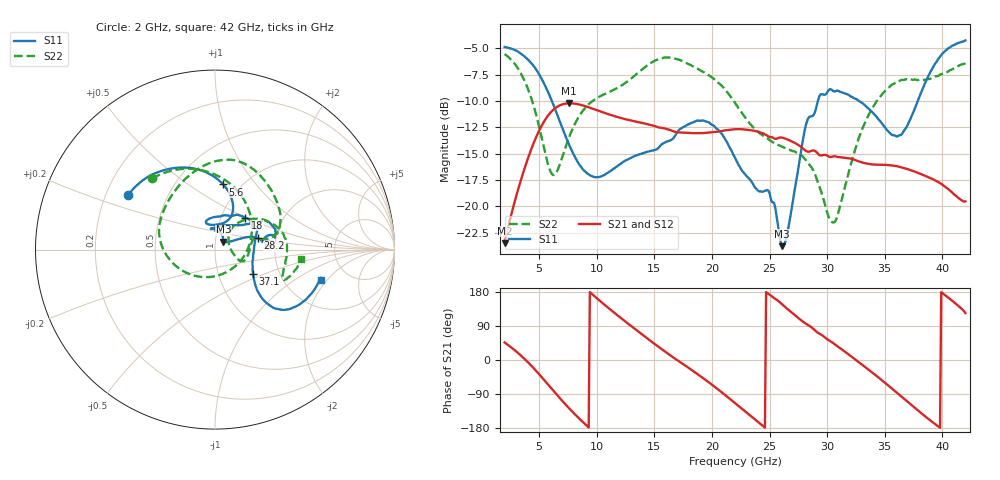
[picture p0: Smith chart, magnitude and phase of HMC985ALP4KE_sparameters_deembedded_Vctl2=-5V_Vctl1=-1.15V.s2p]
!s2p File: Measurements: S11, S21, S12, S22
# GHz S dB R 50.0
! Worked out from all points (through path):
!   401 points, 2 GHz to 42 GHz, reference 50 ohm
!   highest |S21| = -10.21 dB at 7.6 GHz (marker M1); lowest = -23.5 dB at 2 GHz (marker M2)
!   lowest |S11| = -23.8 dB at 26.1 GHz (marker M3), VSWR 1.14, Z = 54.7 + j4.89 ohm
!   |S11| at or under -10 dB: 6.108 GHz to 29.19 GHz (23.08 GHz wide, 131 % of centre); 32.77 GHz to 37.86 GHz (5.089 GHz wide, 14.4 % of centre)
!   |S22| runs from -21.5 to -5.5 dB; largest |S21 - S12| = 0.00035
!   S11 on the Smith chart (normalised r, x): 2 GHz: 0.29, +0.27; 5.6 GHz: 0.83, +0.70; 18 GHz: 1.30, +0.49; 28.2 GHz: 1.61, +0.22; 37.1 GHz: 1.46, -0.42; 42 GHz: 3.18, -1.71
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2  -4.85 147.8  -23.49 46.3  -23.50 46.3  -5.53 131.5
3.6  -5.65 121.3  -16.85 6.5  -16.86 6.5  -7.78 87.0
4.7  -6.94 100.3  -13.52 -27.5  -13.53 -27.5  -11.14 45.1
5.6  -8.73 82.9  -11.64 -58.6  -11.65 -58.6  -15.30 -7.3
6.4  -10.81 70.5  -10.66 -87.0  -10.67 -87.0  -16.94 -74.7
7.6  -14.15 64.4  -10.21 -127.5  -10.21 -127.5  -13.43 -145.6
8.7  -16.35 74.0  -10.38 -161.1  -10.39 -161.1  -11.06 -176.8
12  -16.01 108.4  -11.58 113.0  -11.58 113.0  -8.62 136.3
15.4  -14.39 79.4  -12.51 34.0  -12.51 34.0  -6.01 85.4
18  -12.18 46.5  -13.02 -21.3  -13.03 -21.3  -6.50 54.3
20  -12.26 36.5  -12.96 -65.3  -12.96 -65.2  -7.75 27.0
22  -15.38 53.0  -12.67 -113.8  -12.68 -113.8  -10.17 11.6
24.9  -18.49 96.1  -13.35 174.5  -13.36 174.6  -13.63 11.0
26.1  -23.78 43.5  -13.47 146.6  -13.48 146.6  -14.33 -1.9
28.2  -12.09 14.8  -14.76 95.0  -14.76 95.0  -15.68 -23.1
28.7  -11.42 9.5  -14.71 84.8  -14.71 84.8  -16.39 -23.6
30.6  -9.08 16.1  -15.24 42.9  -15.24 42.9  -21.51 21.0
33  -10.14 31.4  -15.82 -11.8  -15.83 -11.8  -12.77 45.5
35.4  -12.97 9.2  -16.09 -69.7  -16.09 -69.7  -8.66 19.7
37.1  -12.00 -32.6  -16.52 -113.3  -16.52 -113.2  -7.94 0.0
39.7  -5.91 -41.6  -17.73 -176.6  -17.73 -176.6  -7.57 -23.9
42  -4.24 -15.8  -19.53 123.8  -19.54 123.8  -6.36 -6.0
